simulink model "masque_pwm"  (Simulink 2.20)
settings: Solver=FixedStepDiscrete  StartTime=0.0  StopTime=100  FixedStep=1  RelTol=1e-3  AbsTol=1e-6

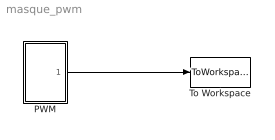
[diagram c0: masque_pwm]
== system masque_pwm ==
  PWM : Subsystem  mask(Masque de génération de signal PWM){T=20, rc=80, vmin=2, vmax=5}
      mask prompts: T "période"; rc "rapport cyclique"; vmin "valeur minimale"; vmax "valeur maximale"
  To Workspace : ToWorkspace  VariableName=pwm  SampleTime=-1
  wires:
  PWM/1(PWM) -> To Workspace/1

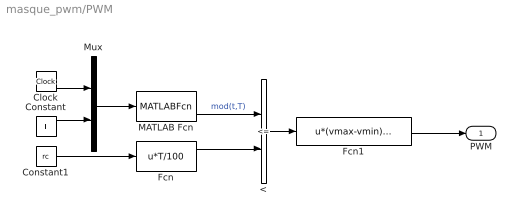
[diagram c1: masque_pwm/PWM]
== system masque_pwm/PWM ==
  < : RelationalOperator  Operator=<=
  Clock : Clock
  Constant : Constant  Value=T
  Constant1 : Constant  Value=rc
  Fcn : Fcn  Expr=u*T/100
  Fcn1 : Fcn  Expr=u*(vmax-vmin)+vmin
  MATLAB Fcn : MATLABFcn  MATLABFcn=mod(u(1),u(2))  OutputWidth=1
  Mux : Mux  Inputs=2
  PWM : Outport  Port=1  InitialOutput=0
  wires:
  Clock/1 -> Mux/1
  Constant/1 -> Mux/2
  Mux/1 -> MATLAB Fcn/1
  Constant1/1 -> Fcn/1
  MATLAB Fcn/1 -> </1  "mod(t,T)"
  Fcn/1 -> </2
  </1 -> Fcn1/1
  Fcn1/1 -> PWM/1
